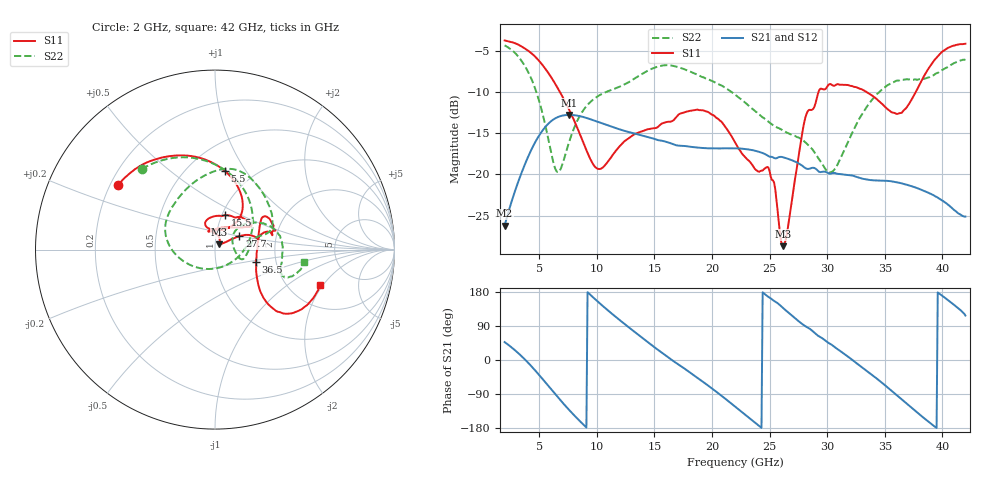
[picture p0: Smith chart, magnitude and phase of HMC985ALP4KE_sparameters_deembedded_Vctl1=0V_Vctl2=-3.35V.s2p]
!s2p File: Measurements: S11, S21, S12, S22
# GHz S dB R 50.0
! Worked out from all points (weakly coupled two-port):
!   401 points, 2 GHz to 42 GHz, reference 50 ohm
!   highest |S21| = -12.78 dB at 7.6 GHz (marker M1); lowest = -26.2 dB at 2 GHz (marker M2)
!   lowest |S11| = -28.7 dB at 26.2 GHz (marker M3), VSWR 1.08, Z = 52.3 + j2.99 ohm
!   |S11| at or under -10 dB: 6.8 GHz to 29.25 GHz (22.45 GHz wide, 125 % of centre); 33.41 GHz to 37.69 GHz (4.283 GHz wide, 12 % of centre)
!   |S22| runs from -19.7 to -4.3 dB; largest |S21 - S12| = 0.00058
!   S11 on the Smith chart (normalised r, x): 2 GHz: 0.23, +0.29; 5.5 GHz: 0.74, +0.81; 15.5 GHz: 1.04, +0.41; 27.7 GHz: 1.30, +0.20; 36.5 GHz: 1.57, -0.23; 42 GHz: 2.94, -1.89
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2  -3.75 146.5  -26.21 47.3  -26.20 47.3  -4.34 132.3
3.6  -4.59 119.3  -19.34 6.3  -19.34 6.3  -6.50 89.6
5.5  -7.12 82.7  -14.30 -57.6  -14.30 -57.6  -13.83 17.3
6.6  -9.50 64.0  -13.06 -97.4  -13.05 -97.4  -19.72 -71.1
7.6  -12.15 53.5  -12.78 -131.8  -12.78 -131.8  -16.07 -145.3
8.7  -15.68 54.1  -12.99 -166.4  -13.00 -166.4  -12.50 -178.8
10.3  -19.34 89.6  -13.72 148.4  -13.70 148.4  -10.35 155.9
12.6  -15.77 109.2  -14.80 90.5  -14.78 90.5  -8.94 122.7
15.4  -14.12 75.2  -15.87 25.0  -15.88 25.0  -6.88 82.7
15.5  -14.00 73.4  -15.88 22.8  -15.90 22.8  -6.85 81.6
19.3  -12.25 33.5  -16.80 -59.2  -16.81 -59.3  -8.24 38.4
22  -16.08 51.7  -16.84 -122.7  -16.83 -122.7  -10.32 17.3
24.9  -19.16 104.3  -17.77 166.5  -17.75 166.5  -13.60 11.0
26.2  -28.70 51.1  -17.93 136.5  -17.93 136.5  -14.71 -3.9
27.7  -16.20 28.8  -18.81 98.1  -18.83 98.0  -15.69 -18.6
28.7  -12.15 12.8  -19.20 77.3  -19.19 77.3  -16.92 -19.0
30.5  -9.22 18.3  -19.83 37.8  -19.84 37.7  -19.61 20.4
33.2  -9.83 34.3  -20.56 -23.2  -20.56 -23.2  -12.32 38.0
35.4  -12.24 11.7  -20.81 -76.3  -20.81 -76.3  -9.06 17.9
36.5  -12.49 -16.6  -21.10 -104.6  -21.10 -104.6  -8.50 6.8
39.5  -5.85 -43.6  -22.73 -179.4  -22.72 -179.4  -7.72 -21.2
42  -4.15 -18.7  -25.11 117.3  -25.12 117.3  -6.03 -7.7
